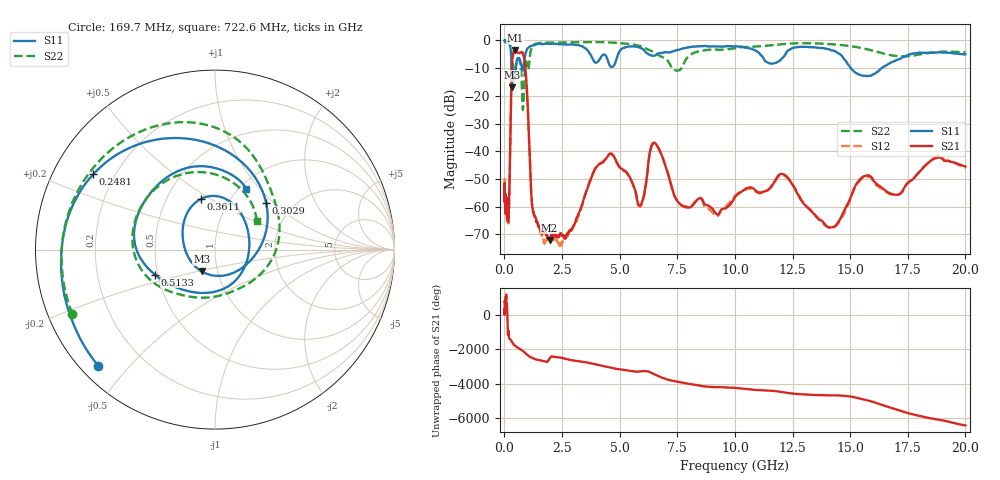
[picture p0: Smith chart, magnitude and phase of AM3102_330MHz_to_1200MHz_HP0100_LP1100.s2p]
! Date/Time: Tue, Sep 11, 2018 5:13 PM
! Network Analyzer: Agilent Technologies E8362B Rev: A.07.50.63
! Sweep from 0.010 to 20.000 GHz, 1601 Points, Sweep Type: LOG
! Power Supply: 4.949 V, 0.001 A
# Hz S DB R 50
!freq MagS11 AngS11 MagS21 AngS21 MagS12 AngS12 MagS22 AngS22
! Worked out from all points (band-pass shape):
!   1601 points, 10 MHz to 20 GHz, reference 50 ohm
!   highest |S21| = -3.53 dB at 473.4 MHz (marker M1); lowest = -72.1 dB at 1.96 GHz (marker M2)
!   |S21| within 3 dB of the highest: 350.1 MHz to 860.2 MHz (510.1 MHz wide, 84.3 % of centre)
!   lowest |S11| = -16.9 dB at 330 MHz (marker M3), VSWR 1.33, Z = 41.9 - j10.4 ohm
!   |S11| at or under -10 dB: 307.9 MHz to 499.3 MHz (191.4 MHz wide, 47.4 % of centre); 759.3 MHz to 821.2 MHz (61.88 MHz wide, 7.83 % of centre); 15.03 GHz to 16.37 GHz (1.347 GHz wide, 8.58 % of centre)
!   |S22| runs from -25.1 to -0.3 dB; largest |S21 - S12| = 0.012
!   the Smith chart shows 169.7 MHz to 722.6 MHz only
!   S11 on the Smith chart (normalised r, x): 169.7 MHz: 0.05, -0.41; 248.1 MHz: 0.12, +0.28; 302.9 MHz: 1.47, +0.90; 361.1 MHz: 0.74, +0.46; 513.3 MHz: 0.48, -0.15; 722.6 MHz: 1.08, +0.85
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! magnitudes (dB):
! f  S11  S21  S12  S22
! 10 MHz  0.0  -57.4  -49.8  -0.3
! 35.55 MHz  0.0  -58.5  -59.3  -0.5
! 126.4 MHz  -0.4  -60.6  -62.0  -1.0
! 169.7 MHz  -0.7  -63.4  -62.9  -1.2
! 248.1 MHz  -2.0  -40.2  -40.0  -1.8
! 302.9 MHz  -8.3  -15.9  -15.9  -3.5
! 330 MHz  -16.9  -8.8  -8.8  -6.0
! 361.1 MHz  -10.7  -5.9  -5.9  -8.3
! 447.2 MHz  -13.5  -3.6  -3.6  -11.4
! 473.4 MHz  -12.1  -3.5  -3.5  -10.4
! 513.3 MHz  -8.8  -3.7  -3.9  -8.3
! 722.6 MHz  -8.4  -4.3  -4.3  -11.0
! 806 MHz  -10.6  -4.7  -4.8  -25.1
! 1.59 GHz  -1.3  -68.9  -69.6  -0.9
! 1.96 GHz  -1.2  -72.1  -71.3  -0.8
! 4.543 GHz  -8.6  -41.2  -41.1  -0.7
! 5.652 GHz  -2.2  -53.6  -53.7  -1.6
! 6.58 GHz  -5.2  -37.4  -37.6  -4.7
! 7.771 GHz  -2.8  -59.9  -59.8  -8.6
! 12.09 GHz  -6.1  -48.3  -48.6  -1.3
! 14.07 GHz  -3.2  -67.5  -67.4  -1.3
! 20 GHz  -5.0  -45.6  -46.2  -4.2
